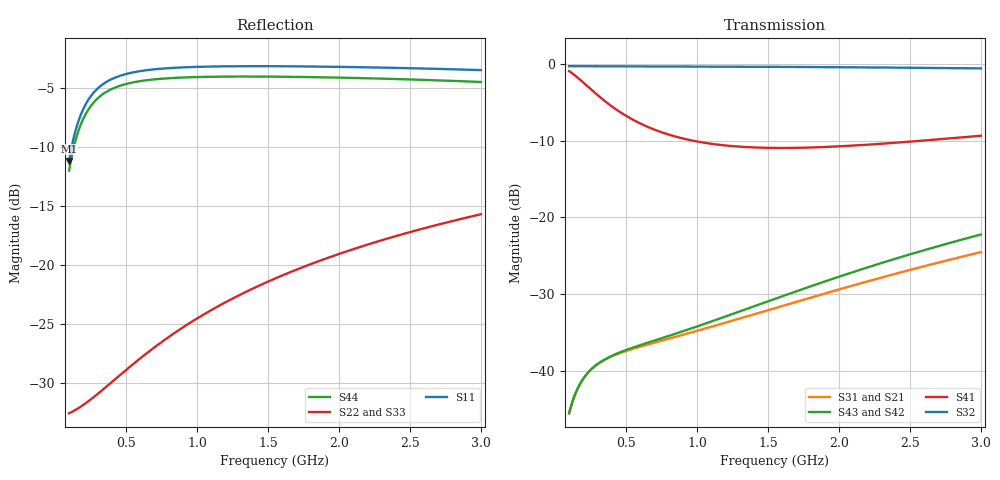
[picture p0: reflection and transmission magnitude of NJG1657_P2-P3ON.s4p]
! NJG1657MD7(1bit control high power DPDT switch) S-parameter
! VDD=2.85V, VCTL(H)=2.6V, VCTL(L)=0V
! P2-P3 ON mode
! Port1...P1, Port2...P2, Port3...P3, Port4...P4
# hz S ma R 50
! 4 Port Network Data from SP1.SP block
! freq  magS11  angS11  magS12  angS12  magS13  angS13  magS14  angS14
!  magS21  angS21  magS22  angS22  magS23  angS23  magS24  angS24
!  magS31  angS31  magS32  angS32  magS33  angS33  magS34  angS34
!  magS41  angS41  magS42  angS42  magS43  angS43  magS44  angS44
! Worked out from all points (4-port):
!   291 points, 100 MHz to 3 GHz, reference 50 ohm
!   strongest paths, dB at 100 MHz, 820 MHz, 1.55 GHz, 2.28 GHz, 3 GHz:
!     S32: -0.3, -0.3, -0.3, -0.4, -0.6
!     S41: -0.9, -9.3, -10.9, -10.4, -9.3
!     S43: -45.6, -35.4, -30.6, -26.1, -22.2
!     S42: -45.6, -35.4, -30.8, -26.3, -22.6
!     S31: -45.6, -35.7, -31.8, -28.0, -24.5
!     S21: -45.6, -35.8, -31.9, -27.9, -24.5
!   lowest |S11| = -11.2 dB at 100 MHz (marker M1), VSWR 1.76, Z = 36.6 - j20.6 ohm
!   |S11| at or under -10 dB: start of sweep to 117.8 MHz
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1e8  0.2764 -109.6  0.005245 66.2  0.005262 66.3  0.9011 -17.1
     0.005245 66.2  0.02344 -14.1  0.9705 -1.4  0.005263 67.0
     0.005262 66.3  0.9705 -1.4  0.02357 -13.9  0.005271 67.0
     0.9011 -17.1  0.005263 67.0  0.005271 67.0  0.2514 -109.9
1.8e8  0.4307 -126.6  0.008242 58.8  0.00827 59.0  0.7878 -27.0
       0.008242 58.8  0.02498 -24.8  0.9701 -2.6  0.008276 60.3
       0.00827 59.0  0.9701 -2.6  0.0251 -24.4  0.008291 60.3
       0.7878 -27.0  0.008276 60.3  0.008291 60.3  0.3914 -127.7
2.9e8  0.5528 -142.2  0.01078 52.1  0.01082 52.4  0.6401 -34.7
       0.01078 52.1  0.02798 -37.6  0.9696 -4.1  0.01085 54.4
       0.01082 52.4  0.9696 -4.1  0.02811 -37.0  0.01087 54.6
       0.6401 -34.7  0.01085 54.4  0.01087 54.6  0.502 -144.2
4.7e8  0.6384 -157.4  0.01307 49.0  0.01312 49.5  0.4795 -38.1
       0.01307 49.0  0.03453 -53.8  0.9688 -6.6  0.01324 52.8
       0.01312 49.5  0.9688 -6.6  0.03468 -52.8  0.01329 52.9
       0.4795 -38.1  0.01324 52.8  0.01329 52.9  0.5792 -160.8
7.2e8  0.6784 -169.3  0.01535 51.7  0.0154 52.4  0.3681 -35.2
       0.01535 51.7  0.04556 -69.3  0.9674 -10.1  0.0158 57.4
       0.0154 52.4  0.9674 -10.1  0.04574 -67.7  0.01592 57.6
       0.3681 -35.2  0.0158 57.4  0.01592 57.6  0.6149 -174.5
1.51e9  0.6976 171.8  0.0249 65.9  0.02494 67.5  0.2843 -19.2
        0.0249 65.9  0.08542 -97.0  0.9613 -21.2  0.02798 75.0
        0.02494 67.5  0.9613 -21.2  0.08561 -93.8  0.02853 74.9
        0.2843 -19.2  0.02798 75.0  0.02853 74.9  0.63 160.9
3e9  0.6715 150.0  0.05981 70.3  0.05934 72.9  0.3411 -10.2
     0.05981 70.3  0.1641 -129.4  0.9385 -42.2  0.07415 77.3
     0.05934 72.9  0.9385 -42.2  0.1631 -123.7  0.07729 76.2
     0.3411 -10.2  0.07415 77.3  0.07729 76.2  0.5978 128.3
